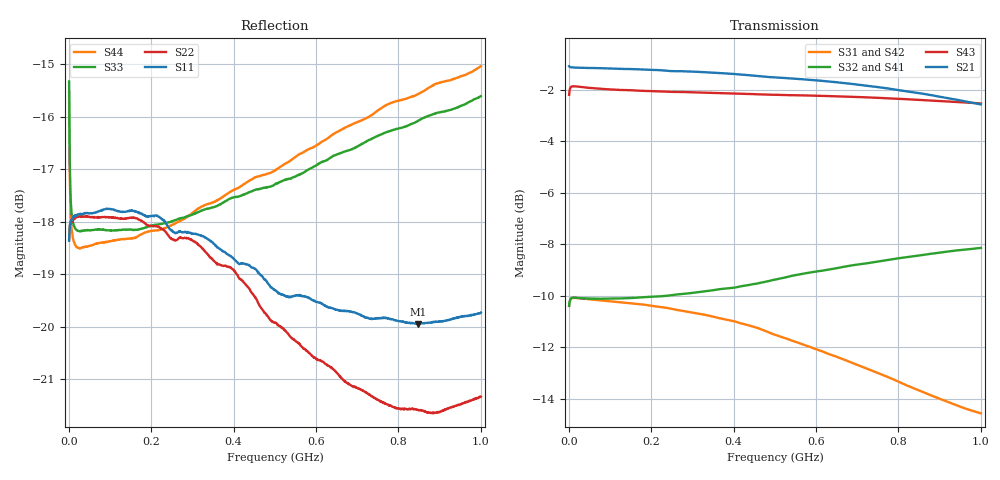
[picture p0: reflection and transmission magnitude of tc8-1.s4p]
!TC8-1, Minicircuits Lab
!unit is from MB29890
!Date: Wednesday, April 11, 2007 16:23:26
!PORT1=PIN6 (primary dot), PORT2=PIN4(primary), PORT3=PIN3(secondary dot), PORT4=PIN1(secondary)
# Hz S  dB  R 50
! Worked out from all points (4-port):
!   1000 points, 1 MHz to 1 GHz, reference 50 ohm
!   strongest paths, dB at 1 MHz, 251 MHz, 501 MHz, 751 MHz, 1 GHz:
!     S21: -1.1, -1.3, -1.5, -1.9, -2.6
!     S43: -2.2, -2.1, -2.2, -2.3, -2.5
!     S32: -10.4, -10.0, -9.4, -8.7, -8.1
!     S41: -10.5, -10.1, -9.5, -8.8, -8.2
!     S31: -10.4, -10.5, -11.5, -13.0, -14.6
!     S42: -10.5, -10.6, -11.6, -13.1, -14.7
!   lowest |S11| = -19.9 dB at 848 MHz (marker M1), VSWR 1.22, Z = 48.8 - j9.92 ohm
!   |S11| at or under -10 dB: start of sweep to end of sweep
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1000000  -18.36 6.1  -1.09 -0.9  -10.38 3.5  -10.49 -176.3
         -1.09 -0.9  -18.33 6.0  -10.38 -176.5  -10.50 3.7
         -10.39 3.5  -10.39 -176.6  -15.33 158.6  -2.21 -176.3
         -10.50 -176.4  -10.50 3.6  -2.20 -176.3  -15.53 158.3
9000000  -17.95 0.8  -1.14 -0.7  -10.07 0.2  -10.16 -179.8
         -1.14 -0.7  -18.01 0.6  -10.07 -179.8  -10.17 0.3
         -10.08 0.2  -10.07 -179.8  -17.95 172.0  -1.88 -180.0
         -10.17 -179.8  -10.16 0.3  -1.87 -180.0  -18.24 171.6
2.9e7  -17.86 -1.0  -1.15 -1.6  -10.09 -1.6  -10.17 178.4
       -1.15 -1.6  -17.90 -1.2  -10.08 178.2  -10.19 -1.7
       -10.10 -1.6  -10.09 178.2  -18.18 172.7  -1.90 177.8
       -10.18 178.4  -10.19 -1.6  -1.89 177.8  -18.50 172.4
4.25e8  -18.80 -31.8  -1.43 -22.0  -11.09 -20.8  -9.72 156.7
        -1.42 -22.0  -19.16 -34.7  -9.60 154.7  -11.19 -21.6
        -11.09 -20.8  -9.61 154.7  -17.49 110.0  -2.18 150.5
        -9.72 156.6  -11.19 -21.7  -2.16 150.5  -17.28 110.0
6.72e8  -19.70 -62.1  -1.76 -34.8  -12.50 -27.9  -9.01 141.6
        -1.75 -34.9  -21.05 -71.2  -8.86 138.4  -12.60 -29.2
        -12.50 -28.0  -8.86 138.4  -16.66 76.9  -2.28 133.8
        -9.01 141.6  -12.61 -29.2  -2.27 133.8  -16.20 80.2
8.48e8  -19.95 -91.2  -2.14 -44.3  -13.66 -29.1  -8.57 130.0
        -2.13 -44.3  -21.58 -107.9  -8.45 125.7  -13.77 -30.4
        -13.65 -29.1  -8.44 125.7  -16.08 53.2  -2.40 121.9
        -8.58 130.0  -13.79 -30.5  -2.40 121.8  -15.57 58.6
1e9  -19.73 -117.0  -2.58 -52.2  -14.55 -26.5  -8.25 119.3
     -2.57 -52.3  -21.33 -143.0  -8.14 114.0  -14.66 -28.2
     -14.55 -26.5  -8.14 114.0  -15.61 32.5  -2.54 111.9
     -8.25 119.2  -14.66 -28.2  -2.54 111.9  -15.04 40.2
